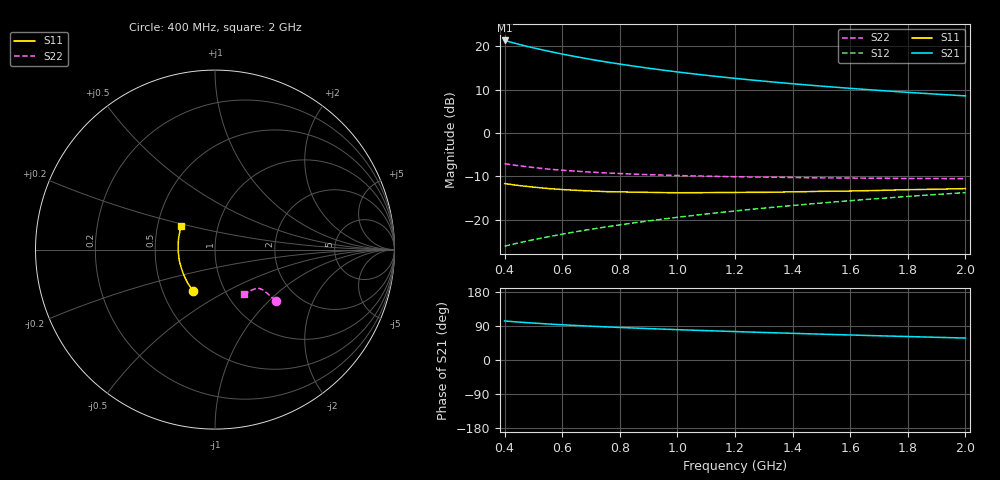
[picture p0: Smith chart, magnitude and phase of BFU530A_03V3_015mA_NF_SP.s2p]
! Filename:  P:\Prog\Test\Noise\ATS_data\Testdata_Net\06 Compressed Noise after Statistics\BFU530A_APG2013_33_A05_03p3V_015mA_NF_CM01_D.sf
! Date/Time: Tue 16/Apr/2013 15:10:56
! BFU530A_APG2013_33_A05_03p3V_1to25mA_NF_CM01_Bias6_R.sf
! Noise Parameter Data File
! BFU530A_APG2013_33_A05_03p3V_1to25mA_NF_CM01
! Date/time: Fri Apr 12 14:21:19 2013
! VAR V_out= 3.300000
! VAR I_out= 14.995000
! VAR V_in= 0.845900
! VAR I_in= 0.166700
! Device data file deembeded for feedlines and parallel
! Original file: \06 Compressed Noise after Statistics\BFU530A_APG2013_33_A05_03p3V_015mA_NF_CM01_R.sf
! Feed-files: PR017V01_150413_Feed1.s2p, PR017V01_150413_Feed2.s2p
! Parallel-file: PR017V01_150413_Par.s2p
# MHz S MA R 50
!  Freq-MHz  S11-mag  S11-arg  S21-mag  S21-arg  S12-mag  S12-arg  S22-mag  S22-arg
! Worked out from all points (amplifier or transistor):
!   37 points, 400 MHz to 2 GHz, reference 50 ohm
!   highest |S21| = 21.4 dB at 400 MHz (marker M1)
!   |S21| within 3 dB of that: start of sweep to 590 MHz
!   unconditionally stable (mu >= 1): 1.049 GHz to end of sweep
!   at 500 MHz: K = 0.89, MSG = 22.2 dB, |S12| = -24.6 dB
!   at 1.1 GHz: K = 1.00, MAG = 15.7 dB, |S12| = -18.7 dB
!   at 2 GHz: K = 1.00, MAG = 10.9 dB, |S12| = -13.8 dB
!   lowest NFmin = 0.89 dB at 420 MHz
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400  0.261 -117.6  11.74 103.1  0.04942 68.5  0.4428 -39.9
420  0.2557 -120.5  11.26 101.8  0.0513 68.7  0.4325 -40.0
440  0.2502 -123.3  10.81 100.6  0.05313 68.9  0.4236 -40.0
460  0.2456 -125.7  10.39 99.5  0.055 69.1  0.4156 -40.1
500  0.2377 -130.8  9.641 97.5  0.05871 69.4  0.4007 -40.0
550  0.2291 -136.7  8.861 95.0  0.06326 69.9  0.3841 -39.9
600  0.2229 -141.6  8.181 93.0  0.06805 70.1  0.3725 -39.9
650  0.218 -146.4  7.601 91.0  0.07279 70.4  0.3628 -40.0
700  0.2144 -150.8  7.097 89.2  0.07753 70.6  0.3544 -40.1
750  0.2109 -155.0  6.654 87.5  0.08231 70.8  0.3469 -40.2
800  0.2095 -158.8  6.267 85.9  0.08712 70.9  0.3413 -40.5
850  0.208 -162.7  5.923 84.3  0.09191 70.9  0.3354 -40.8
900  0.2066 -166.2  5.613 82.9  0.09676 70.9  0.3308 -41.1
950  0.2056 -169.4  5.335 81.5  0.1016 70.9  0.3272 -41.5
1050  0.2049 -175.4  4.855 78.8  0.1114 70.8  0.3206 -42.3
1150  0.206 179.0  4.459 76.2  0.1212 70.5  0.3152 -43.4
1200  0.2061 176.5  4.286 75.0  0.1261 70.3  0.3134 -44.0
1350  0.208 169.3  3.841 71.5  0.1408 69.7  0.3086 -46.0
1500  0.2126 162.8  3.486 68.2  0.1557 68.9  0.304 -48.2
1650  0.2161 157.1  3.196 65.0  0.1707 68.0  0.3017 -50.7
1750  0.2199 153.4  3.029 62.9  0.1805 67.4  0.2998 -52.4
2000  0.2287 145.4  2.689 57.9  0.2053 65.6  0.2976 -57.2
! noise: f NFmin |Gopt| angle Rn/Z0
400  0.9315  0.1946  -171.5  0.0808
460  0.9144  0.1968  -170.3  0.0757
600  0.9925  0.1906  -156.8  0.0945
800  0.9732  0.222  -160.2  0.0772
1000  0.9993  0.2437  -160.1  0.0729
1200  1.016  0.2473  -151  0.0827
1400  1.052  0.2618  -147.4  0.0894
1600  1.071  0.2899  -140.7  0.0871
1800  1.063  0.333  -139.3  0.0799
2000  1.112  0.3437  -132  0.0898
